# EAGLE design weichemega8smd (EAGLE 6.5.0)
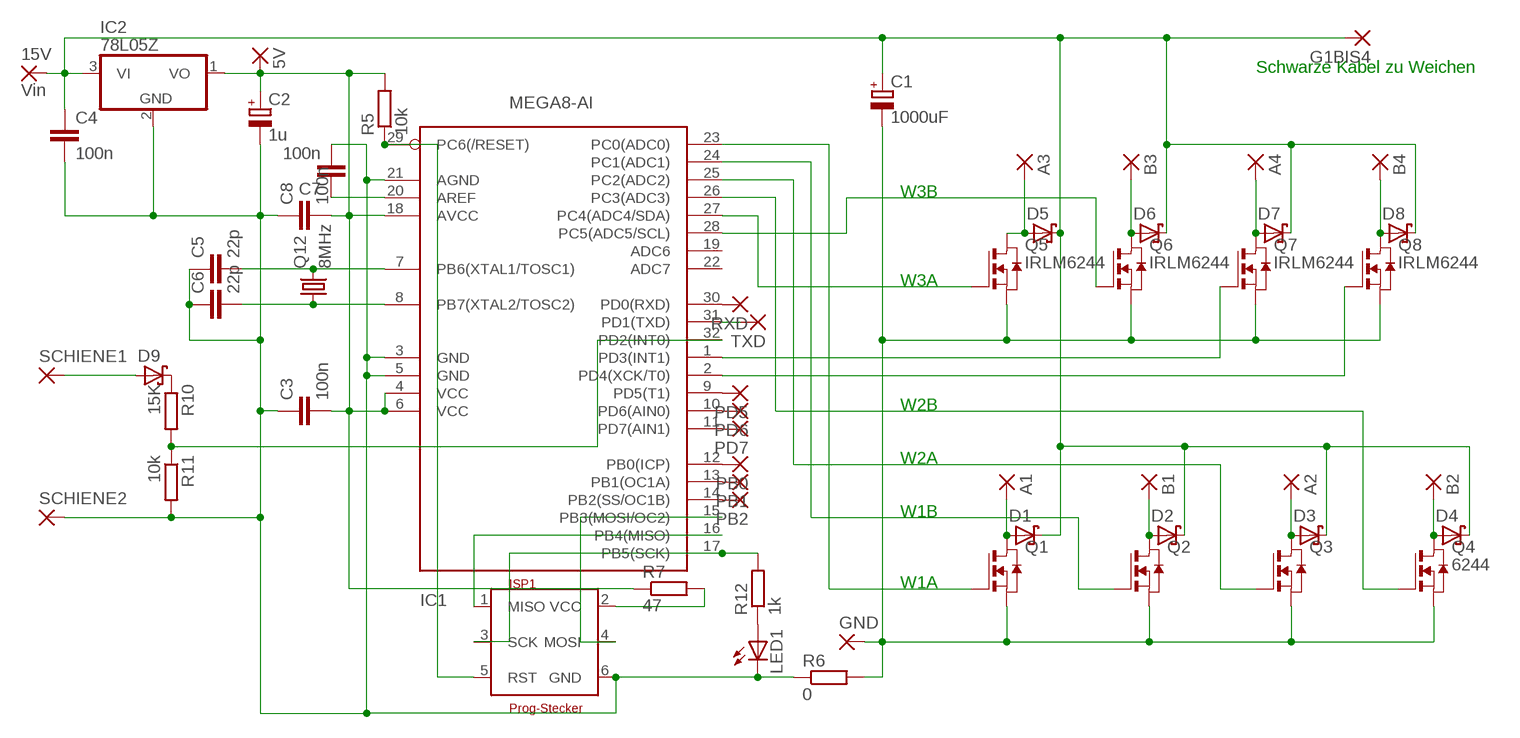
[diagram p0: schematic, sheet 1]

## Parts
5V  2,15/1,0  [2,15/1,0]
15V  Vin  2,15/1,0  [2,15/1,0]
A1  2,15/1,0  [2,15/1,0]
A2  2,15/1,0  [2,15/1,0]
A3  2,15/1,0  [2,15/1,0]
A4  2,15/1,0  [2,15/1,0]
B1  2,15/1,0  [2,15/1,0]
B2  2,15/1,0  [2,15/1,0]
B3  2,15/1,0  [2,15/1,0]
B4  2,15/1,0  [2,15/1,0]
C1  1000uF  CPOL-EUE2.5-7  [E2,5-7]
C2  1u  CPOL-EUE2.5-5  [E2,5-5]
C3  100n  C-EU025-024X044  [C025-024X044]
C4  100n  C-EU025-024X044  [C025-024X044]
C5  22p  C-EU025-024X044  [C025-024X044]
C6  22p  C-EU025-024X044  [C025-024X044]
C7  100n  C-EU025-024X044  [C025-024X044]
C8  100n  C-EU025-024X044  [C025-024X044]
D1  SCHOTTKY-DIODESMD  [SMB]
D2  SCHOTTKY-DIODESMD  [SMB]
D3  SCHOTTKY-DIODESMD  [SMB]
D4  SCHOTTKY-DIODESMD  [SMB]
D5  SCHOTTKY-DIODESMD  [SMB]
D6  SCHOTTKY-DIODESMD  [SMB]
D7  SCHOTTKY-DIODESMD  [SMB]
D8  SCHOTTKY-DIODESMD  [SMB]
D9  SCHOTTKY-DIODESMD  [SMB]
G1BIS4  2,15/1,0  [2,15/1,0]
GND  2,15/1,0  [2,15/1,0]
IC1  MEGA8-AI  [TQFP32-08]
IC2  78L05Z  [TO92]
ISP1  Prog-Stecker  ISP6N  [ISP6]
LED1  TLLG4400  [LED3MM]
PB0  1,6/0,8  [1,6/0,8]
PB1  1,6/0,8  [1,6/0,8]
PB2  1,6/0,8  [1,6/0,8]
PD5  1,6/0,8  [1,6/0,8]
PD6  1,6/0,8  [1,6/0,8]
PD7  1,6/0,8  [1,6/0,8]
Q1  NMOSSOT23  [SOT-23]
Q2  NMOSSOT23  [SOT-23]
Q3  NMOSSOT23  [SOT-23]
Q4  6244  NMOSSOT23  [SOT-23]
Q5  IRLM6244  NMOSSOT23  [SOT-23]
Q6  IRLM6244  NMOSSOT23  [SOT-23]
Q7  IRLM6244  NMOSSOT23  [SOT-23]
Q8  IRLM6244  NMOSSOT23  [SOT-23]
Q12  8MHz  CRYSTALTC26V  [TC26V]
R5  10k  R-EU_M1406  [M1406]
R6  0  R-EU_0204/5  [0204/5]
R7  47  R-EU_0204/5  [0204/5]
R10  15K  R-EU_M1406  [M1406]
R11  10k  R-EU_M1406  [M1406]
R12  1k  R-EU_0204/2V  [0204V]
RXD  1,6/0,8  [1,6/0,8]
SCHIENE1  2,15/1,0  [2,15/1,0]
SCHIENE2  2,15/1,0  [2,15/1,0]
TXD  1,6/0,8  [1,6/0,8]

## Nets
GND [dick]: C2.- C3.1 C4.2 C5.1 C6.1 C7.2 C8.1 IC1.3(GND) IC1.5(GND) IC1.21(AGND) IC2.2(GND) ISP1.6(GND) LED1.K(C) R6.1 R11.2 SCHIENE2.1(P)
GND1 [dick3]: C1.- GND.1(P) Q1.2(S) Q2.2(S) Q3.2(S) Q4.2(S) Q5.2(S) Q6.2(S) Q7.2(S) Q8.2(S) R6.2
N$1: IC1.23(PC0(ADC0)) Q1.3(G)
N$2: IC1.26(PC3(ADC3)) Q4.3(G)
N$3: IC1.24(PC1(ADC1)) Q2.3(G)
N$4: IC1.25(PC2(ADC2)) Q3.3(G)
N$5: IC1.28(PC5(ADC5/SCL)) Q6.3(G)
N$6: IC1.16(PB4(MISO)) ISP1.1(MISO)
N$7 [dick2]: B2.1(P) D4.A Q4.1(D)
N$8: IC1.10(PD6(AIN0)) PD6.1(P)
N$9: IC1.29(PC6(/RESET)) ISP1.5(RST) R5.1
N$10 [dick2]: A1.1(P) D1.A Q1.1(D)
N$11 [dick2]: B1.1(P) D2.A Q2.1(D)
N$12 [dick2]: A2.1(P) D3.A Q3.1(D)
N$13 [dick2]: A4.1(P) D7.A Q7.1(D)
N$14: IC1.15(PB3(MOSI/OC2)) ISP1.4(MOSI)
N$15 [dick2]: A3.1(P) D5.A Q5.1(D)
N$16 [dick2]: B3.1(P) D6.A Q6.1(D)
N$17: LED1.A R12.1
N$18: IC1.17(PB5(SCK)) ISP1.3(SCK) R12.2
N$19: IC1.11(PD7(AIN1)) PD7.1(P)
N$20 [dick2]: D9.C R10.1
N$21: C5.2 IC1.7(PB6(XTAL1/TOSC1)) Q12.2
N$22: C6.2 IC1.8(PB7(XTAL2/TOSC2)) Q12.1
N$23 [dick]: ISP1.2(VCC) R7.2
N$24 [dick2]: D9.A SCHIENE1.1(P)
N$25: IC1.32(PD2(INT0)) R10.2 R11.1
N$26 [dick2]: B4.1(P) D8.A Q8.1(D)
N$27: C7.1 IC1.20(AREF)
N$28: IC1.30(PD0(RXD)) RXD.1(P)
N$29: IC1.31(PD1(TXD)) TXD.1(P)
N$30: IC1.12(PB0(ICP)) PB0.1(P)
N$31: IC1.13(PB1(OC1A)) PB1.1(P)
N$32: IC1.14(PB2(SS/OC1B)) PB2.1(P)
N$33: IC1.27(PC4(ADC4/SDA)) Q5.3(G)
N$34: IC1.1(PD3(INT1)) Q7.3(G)
N$35: IC1.2(PD4(XCK/T0)) Q8.3(G)
N$36: IC1.9(PD5(T1)) PD5.1(P)
VCC [dick]: 5V.1(P) C2.+ C3.2 C8.2 IC1.4(VCC) IC1.6(VCC) IC1.18(AVCC) IC2.1(VO) R5.2 R7.1
VIN [dick3]: 15V.1(P) C1.+ C4.1 D1.C D2.C D3.C D4.C D5.C D6.C D7.C D8.C G1BIS4.1(P) IC2.3(VI)
Unconnected: IC1.19(ADC6) IC1.22(ADC7)

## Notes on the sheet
- Schwarze Kabel zu Weichen
- W3B
- W3A
- W2B
- W2A
- W1B
- W1A

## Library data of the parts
5V 15V A1-A4 B1-B4 G1BIS4 GND SCHIENE1 SCHIENE2 = wirepad:2,15/1,0: THROUGH-HOLE PAD
C1 C2 = rcl:CPOL-EU: POLARIZED CAPACITOR, European symbol
C3-C8 = rcl:C-EU: CAPACITOR, European symbol
D1-D9 = diode:SCHOTTKY-DIODE: Schottky Diode
IC1 = avr-7:MEGA8: MICROCONTROLLER 8 Kbytes FLASH 1 kbytes SRAM 512 bytes EEPROM USART 6-channel 10 bit ADC 2-channel 8 bit ADC
IC2 = linear:78*: Positive VOLTAGE REGULATOR Source: http://cache.national.com/ds/LM/LM78L05.pdf http://www.fairchildsemi.com/ds/LM/LM7805.pdf
ISP1 = 6_stecker:ISP6: ISP-Stecker 6polig
LED1 = led:TLLG4400: Low Current (2mA) LED 3 mm Tinted Diffused Package color GREEN; MF: VISHAY SEMICONDUCTOR; OC_FARNELL: 1612435
PB0 PB1 PB2 PD5-PD7 RXD TXD = wirepad:1,6/0,8: THROUGH-HOLE PAD
Q1-Q8 = zetex:NMOSSOT23: MOS FET; OC_FARNELL: unknown; OC_NEWARK: unknown
Q12 = crystal:CRYSTAL: CRYSTAL; OC_FARNELL: unknown; OC_NEWARK: unknown
R5-R7 R10-R12 = rcl:R-EU_: RESISTOR, European symbol

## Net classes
0 default: width 0.254 mm
1 dick: width 0.406 mm
2 dick2: width 0.813 mm
3 dick3: width 1.016 mm

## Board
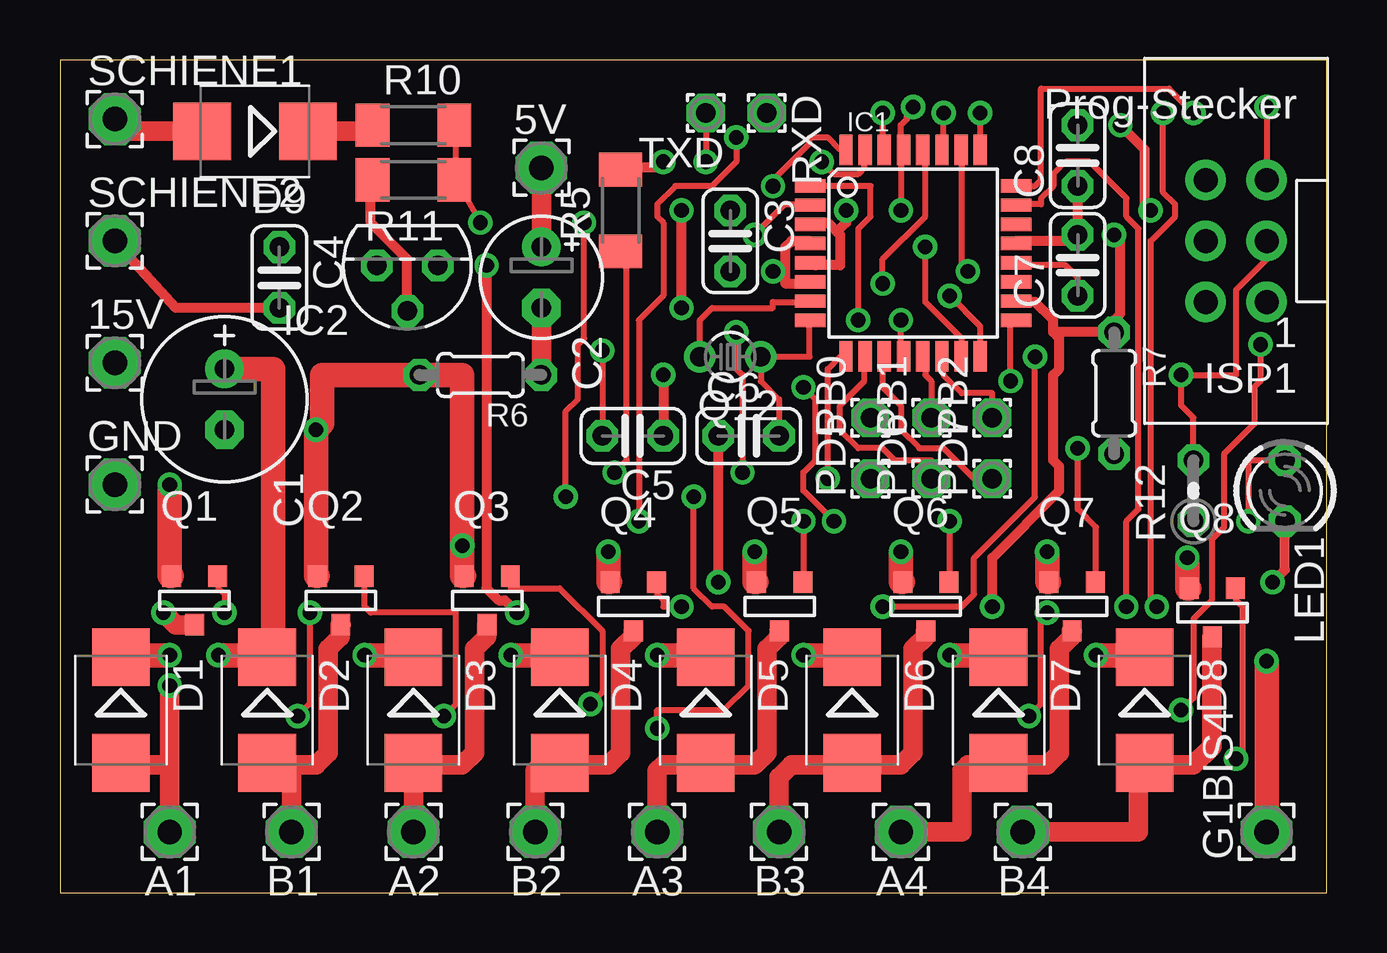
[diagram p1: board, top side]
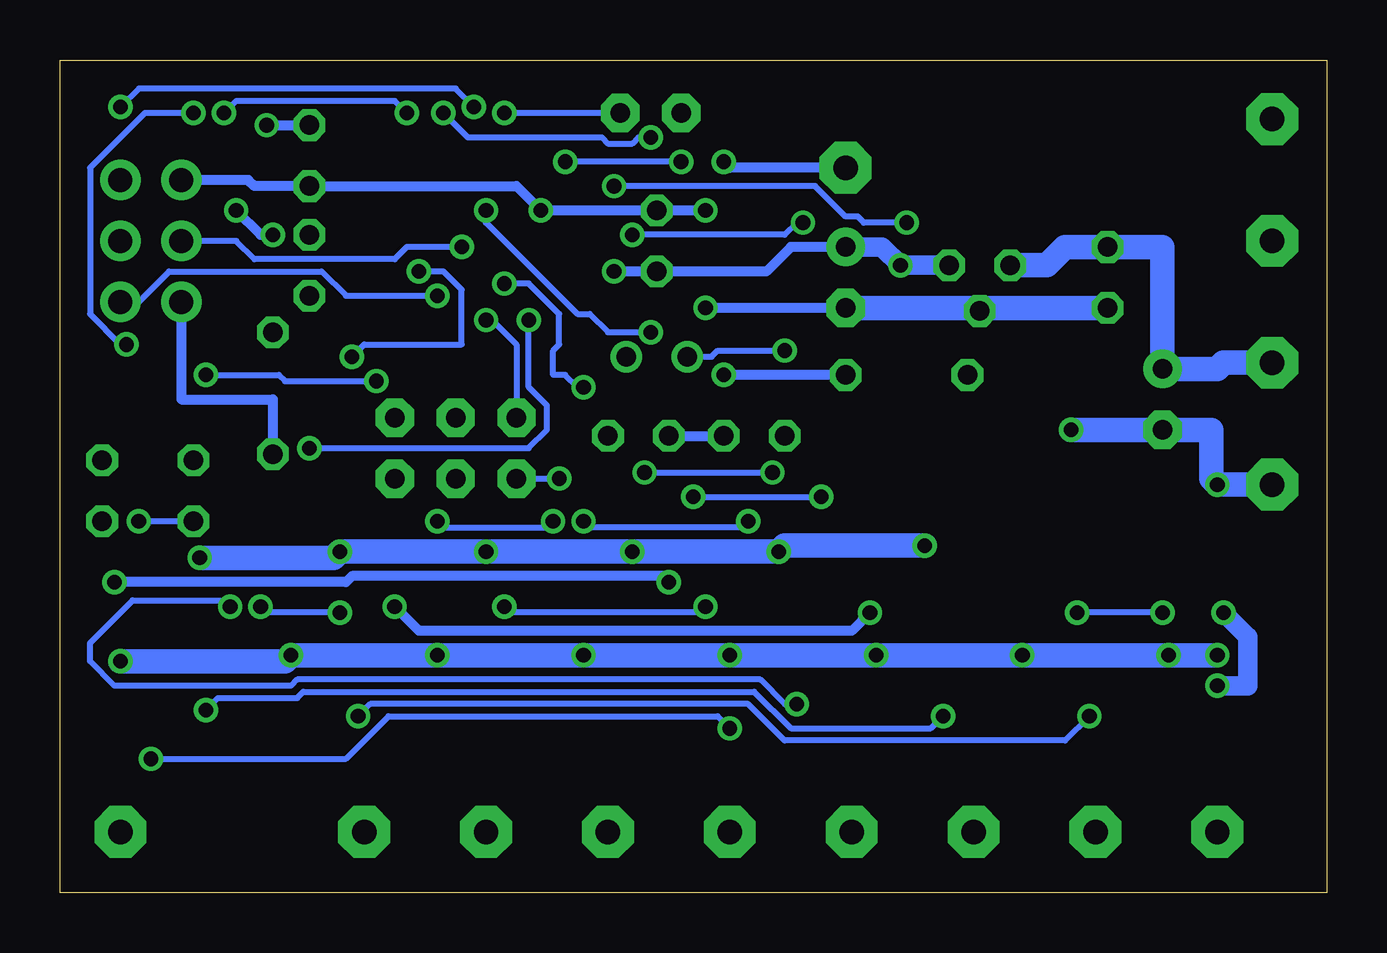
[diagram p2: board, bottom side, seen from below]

Size 52.81 x 34.72 mm. Coordinates in mm from the lower left corner, seen from the top.
Outline: 0,0 52.81,0 52.81,34.72 0,34.72 0,0
Copper layers (1*16): Top 0.035mm / dielectric 1.5mm / Bottom 0.035mm
Design rules "default": minimum track width 10mil, minimum drill 24mil, track to track 8mil, track to pad 8mil, pad to pad 8mil, via to via 8mil, smd to smd 8mil, copper to edge 40mil, drill to drill 8mil, minimum pad ring 10mil, minimum via ring 8mil, stop-mask expansion 4mil, vias tented up to drill 0mil, thermal gap 10mil

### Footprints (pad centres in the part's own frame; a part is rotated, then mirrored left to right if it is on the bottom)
2,15/1,0 = drill 1.016 pad 2.159 octagon: 1 0,0
E2,5-7 = drill 0.813 pad 1.6: + -1.27,0 | drill 0.813 pad 1.6 octagon: - 1.27,0
E2,5-5 = drill 0.813 pad 1.6: + -1.27,0 | drill 0.813 pad 1.6 octagon: - 1.27,0
C025-024X044 = drill 0.813 octagon: 1 -1.27,0; 2 1.27,0
SMB = smd 2.4 x 2.4: A 2.2,0; C -2.2,0
TQFP32-08 = smd 1.27 x 0.559: 1 -4.293,2.8; 2 -4.293,2; 3 -4.293,1.2; 4 -4.293,0.4; 5 -4.293,-0.4; 6 -4.293,-1.2; 7 -4.293,-2; 8 -4.293,-2.8; 17 4.293,-2.8; 18 4.293,-2; 19 4.293,-1.2; 20 4.293,-0.4; 21 4.293,0.4; 22 4.293,1.2; 23 4.293,2; 24 4.293,2.8 | smd 0.559 x 1.27: 9 -2.8,-4.293; 10 -2,-4.293; 11 -1.2,-4.293; 12 -0.4,-4.293; 13 0.4,-4.293; 14 1.2,-4.293; 15 2,-4.293; 16 2.8,-4.293; 25 2.8,4.293; 26 2,4.293; 27 1.2,4.293; 28 0.4,4.293; 29 -0.4,4.293; 30 -1.2,4.293; 31 -2,4.293; 32 -2.8,4.293
TO92 = drill 0.813 octagon: 1 -1.27,0; 2 0,1.905; 3 1.27,0
ISP6 = drill 1 pad 1.676: 1 -1.27,2.54; 2 1.27,2.54; 3 -1.27,0; 4 1.27,0; 5 -1.27,-2.54; 6 1.27,-2.54
LED3MM = drill 0.813 octagon: A -1.27,0; K 1.27,0
1,6/0,8 = drill 0.813 pad 1.6 octagon: 1 0,0
SOT-23 = smd 0.787 x 0.889: 1 0.025,-1.016; 2 -0.94,1.016; 3 0.991,1.016
TC26V = drill 0.813: 1 -1.27,0; 2 1.27,0
M1406 = smd 1.4 x 1.8: 1 -1.7,0; 2 1.7,0
0204/5 = drill 0.813 octagon: 1 -2.54,0; 2 2.54,0
0204V = drill 0.813 octagon: 1 -1.27,0; 2 1.27,0

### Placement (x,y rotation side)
5V  20.07,30.23 0 top
15V  2.29,22.1 0 top
A1  4.57,2.54 180 top
A2  14.73,2.54 180 top
A3  24.89,2.54 180 top
A4  35.05,2.54 180 top
B1  9.65,2.54 180 top
B2  19.81,2.54 180 top
B3  29.97,2.54 180 top
B4  40.13,2.54 180 top
C1  6.86,20.57 270 top
C2  20.07,25.65 270 top
C3  27.94,27.18 270 top
C4  9.14,25.65 270 top
C5  23.88,19.05 180 top
C6  28.7,19.05 0 top
C7  42.42,26.16 90 top
C8  42.42,30.73 90 top
D1  2.54,7.62 270 top
D2  8.64,7.62 270 top
D3  14.73,7.62 270 top
D4  20.83,7.62 270 top
D5  26.92,7.62 270 top
D6  33.02,7.62 270 top
D7  39.12,7.62 270 top
D8  45.21,7.62 270 top
D9  8.13,31.75 180 top
G1BIS4  50.29,2.54 90 top
GND  2.29,17.02 0 top
IC1  35.56,26.67 0 top
IC2  14.48,26.16 180 top
ISP1  49.02,27.18 180 top
LED1  51.05,16.76 270 top
PB0  33.78,19.81 90 top
PB1  36.32,19.81 90 top
PB2  38.86,19.81 90 top
PD5  33.78,17.27 90 top
PD6  36.32,17.27 90 top
PD7  38.86,17.27 90 top
Q1  5.59,12.19 0 top
Q2  11.68,12.19 0 top
Q3  17.78,12.19 0 top
Q4  23.88,11.94 0 top
Q5  29.97,11.94 0 top
Q6  36.07,11.94 0 top
Q7  42.16,11.94 0 top
Q8  48.01,11.68 0 top
Q12  27.94,22.35 180 top
R5  23.37,28.45 90 top
R6  17.53,21.59 180 top
R7  43.94,20.83 270 top
R10  14.73,32 0 top
R11  14.73,29.72 180 top
R12  47.24,16.76 90 top
RXD  29.46,32.51 270 top
SCHIENE1  2.29,32.26 0 top
SCHIENE2  2.29,27.18 0 top
TXD  26.92,32.51 180 top

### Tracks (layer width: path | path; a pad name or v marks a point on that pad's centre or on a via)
GND  (via drill 0.61)
  Top 0.406: LED1.K 51.05,13.46 v50.55,12.95 | C6.1 v27.43,12.95 | 32.38,27.56 32,27.94 31.5,27.94 IC1.3 | 32.38,27.56 32.51,27.43 32.51,26.16 31.5,26.16 IC1.5 | 32.38,27.56 32.77,27.94 v32.77,28.45 | IC1.21 39.88,27.18 42.42,27.18 C7.2 C8.1 | IC2.2 14.48,26.42 12.95,27.94 12.95,29.72 R11.2 | SCHIENE2.1 4.83,24.38 C4.2 | v25.91,24.38 v25.91,28.45 | v25.15,21.59 C5.1
  Top 0.813: C2.- R6.1
  Bottom 0.406: C6.1 C5.1 | v50.55,12.95 40.89,12.95 40.64,13.21 27.69,13.21 v27.43,12.95 | ISP1.6 44.96,29.72 44.7,29.46 C8.1 33.78,29.46 v32.77,28.45 C3.1 v25.91,28.45 | 14.48,24.38 IC2.2 | C2.- v25.91,24.38 | R6.1 v25.15,21.59
  Bottom 1.016: C4.2 14.48,24.38 C2.-
GND1  (via drill 0.61)
  Top 1.016: v22.86,14.22 22.86,12.95 Q4.2 | v28.96,14.22 28.96,12.95 Q5.2 | v35.05,14.22 35.05,12.95 Q6.2 | v41.15,14.22 41.15,12.95 Q7.2 | v46.99,13.97 46.99,12.7 Q8.2 | Q3.2 16.76,13.21 v16.76,14.48 16.76,21.59 R6.2 10.92,21.59 10.92,19.56 v10.67,19.3 10.67,13.21 Q2.2 | v4.57,17.02 4.57,13.21 Q1.2
  Bottom 1.016: v46.99,13.97 41.4,13.97 v41.15,14.22 v35.05,14.22 v28.96,14.22 v22.86,14.22 22.61,14.48 v16.76,14.48 | GND.1 v4.57,17.02 4.83,17.27 4.83,19.3 C1.- v10.67,19.3
N$1  (via drill 0.61)
  Top 0.254: v44.45,11.94 44.45,15.49 44.96,16 44.96,27.69 44.45,28.19 44.45,28.96 42.93,30.48 41.91,30.48 41.4,29.97 41.4,29.46 40.89,28.96 40.89,28.7 39.88,28.7 IC1.23 | v41.15,11.68 40.89,11.43 40.89,7.87 v40.39,7.37 | v9.91,7.37 10.41,7.87 v10.41,11.68 | v6.86,11.68 6.86,12.45 6.6,12.7 6.6,13.21 Q1.3
  Bottom 0.254: v44.45,11.94 44.2,11.68 v41.15,11.68 | v40.39,7.37 39.88,7.87 24.13,7.87 22.61,6.35 10.92,6.35 v9.91,7.37 | v6.86,11.68 v10.41,11.68
N$2  (via drill 0.61)
  Top 0.254: v37.85,25.91 37.59,26.16 37.59,30.73 IC1.26 | v40.64,22.35 40.64,16.51 38.1,13.97 38.1,12.45 37.59,11.94 v34.29,11.94 | v25.91,11.94 25.15,11.94 25.15,12.19 24.89,12.45 24.89,12.95 Q4.3
  Bottom 0.254: v37.85,25.91 36.83,25.91 36.07,25.15 36.07,22.86 40.13,22.86 v40.64,22.35 | v34.29,11.94 34.04,11.68 26.16,11.68 v25.91,11.94
N$3  (via drill 0.61)
  Top 0.254: v16,7.37 16.51,7.87 16.51,11.68 12.95,11.68 12.7,11.94 12.7,13.21 Q2.3 | v46.74,7.62 47.24,8.13 47.24,11.43 48.01,12.19 48.01,14.73 48.51,15.24 48.51,18.29 49.78,19.56 49.78,21.08 50.04,21.34 v50.04,22.86 | v47.24,32.51 46.23,33.53 40.89,33.53 40.89,29.72 40.64,29.46 39.88,29.46 IC1.24
  Bottom 0.254: v16,7.37 16.51,6.86 22.35,6.86 23.88,8.38 42.67,8.38 42.93,8.13 46.23,8.13 v46.74,7.62 | v50.04,22.86 50.29,22.86 51.56,24.13 51.56,30.23 49.28,32.51 v47.24,32.51
N$4  (via drill 0.61)
  Top 0.254: v38.35,32.51 38.35,30.99 IC1.25 | v45.97,32.51 45.97,29.21 46.48,28.7 46.48,28.19 45.47,27.18 45.47,12.19 v45.72,11.94 | v22.1,7.87 22.61,8.38 22.61,10.92 20.83,12.7 18.8,12.7 18.8,13.21 Q3.3
  Bottom 0.254: v38.35,32.51 38.86,33.02 45.47,33.02 v45.97,32.51 | v45.72,11.94 45.97,12.19 49.78,12.19 51.56,10.41 51.56,9.65 50.55,8.64 43.18,8.64 42.93,8.89 23.62,8.89 22.61,7.87 v22.1,7.87
N$5  (via drill 0.61)
  Top 0.254: v34.29,25.4 34.29,26.42 36.07,28.19 36.07,30.73 IC1.28 | v30.99,21.08 31.5,20.57 31.5,18.03 30.99,17.53 30.99,16.76 v32.26,15.49 | v37.08,15.49 37.08,12.95 Q6.3
  Bottom 0.254: v34.29,25.4 33.27,25.4 32,24.13 32,22.86 32.26,22.61 32.26,21.59 31.75,21.59 31.24,21.08 v30.99,21.08 | v32.26,15.49 32.51,15.24 36.83,15.24 v37.08,15.49
N$6  (via drill 0.61)
  Top 0.254: v37.08,24.89 38.35,23.62 38.35,22.61 IC1.16
  Bottom 0.254: v37.08,24.89 40.89,24.89 41.91,25.91 48.26,25.91 49.53,24.64 ISP1.1
N$7
  Top 0.813: Q4.1 23.88,10.92 23.88,10.67 23.37,10.16 23.37,5.84 22.86,5.33 20.83,5.33 D4.A 20.57,5.33 20.07,5.33 19.81,5.08 B2.1
N$8
  Top 0.254: PD6.1 36.32,18.03 34.8,18.03 34.29,18.54 33.27,18.54 32.51,19.3 32.51,20.32 33.53,21.34 33.53,22.35 IC1.10
N$9  (via drill 0.61)
  Top 0.254: v50.29,32.77 ISP1.5 | v35.56,32.77 35.31,32.51 35.31,32.26 35.05,32 35.05,30.99 IC1.29 35.05,30.73 v35.05,28.45 | v23.11,17.53 23.62,18.03 23.62,26.67 23.37,26.67 R5.1 | v28.45,17.53 28.45,21.59 28.19,21.84 v28.19,23.37
  Bottom 0.254: v50.29,32.77 49.53,33.53 36.32,33.53 v35.56,32.77 | v28.45,17.53 v23.11,17.53 | v28.19,23.37 29.97,23.37 30.73,24.13 31.24,24.13 35.05,27.94 v35.05,28.45
N$10  (via drill 0.61)
  Top 0.813: Q1.1 4.83,11.18 v4.32,11.68 | A1.1 4.57,5.33 | 4.57,5.33 v4.57,8.64 | 4.57,5.33 2.54,5.33 D1.A
  Bottom 0.813: v4.32,11.68 3.3,10.67 3.3,8.64 v4.57,8.64
N$11
  Top 0.813: Q2.1 11.68,11.18 11.68,10.67 11.18,10.16 11.18,5.84 10.67,5.33 8.64,5.33 D2.A 9.65,5.08 B1.1
N$12
  Top 0.813: Q3.1 17.78,11.18 17.78,10.67 17.27,10.16 17.27,5.84 16.76,5.33 14.73,5.33 D3.A A2.1
N$13
  Top 0.813: Q7.1 42.16,10.92 42.16,10.67 41.66,10.16 41.66,5.84 41.15,5.33 39.12,5.33 D7.A 38.86,5.33 37.85,5.33 37.59,5.08 37.59,2.54 A4.1
N$14  (via drill 0.61)
  Top 0.254: v36.07,26.92 36.07,24.64 37.59,23.11 37.59,22.61 IC1.15
  Bottom 0.254: ISP1.4 45.47,27.18 44.7,26.42 38.86,26.42 38.35,26.92 v36.07,26.92
N$15
  Top 0.813: Q5.1 29.97,10.92 29.97,10.67 29.46,10.16 29.46,5.84 28.96,5.33 26.92,5.33 D5.A 26.67,5.33 25.15,5.33 24.89,5.08 A3.1
N$16
  Top 0.813: Q6.1 36.07,10.92 36.07,10.67 35.56,10.16 35.56,5.84 35.05,5.33 33.02,5.33 D6.A 32.77,5.33 30.48,5.33 29.97,4.83 B3.1
N$17  (via drill 0.61)
  Top 0.254: v49.53,15.49 49.53,18.03 LED1.A
  Bottom 0.254: v49.53,15.49 R12.1
N$18  (via drill 0.61)
  Top 0.254: v39.62,21.34 39.62,23.62 IC1.17 | R12.2 47.24,19.81 46.74,20.32 v46.74,21.59 49.02,21.59 49.02,25.15 50.29,26.42 ISP1.3
  Bottom 0.254: v39.62,21.34 43.43,21.34 43.69,21.59 v46.74,21.59
N$19
  Top 0.254: PD7.1 38.1,17.27 36.83,18.54 35.81,18.54 35.05,19.3 35.05,20.32 34.29,21.08 34.29,22.35 IC1.11
N$20
  Top 0.813: R10.1 12.7,32 12.45,31.75 D9.C
N$21  (via drill 0.61)
  Top 0.254: Q12.2 26.67,23.88 27.18,24.38 29.72,24.38 29.72,24.64 31.24,24.64 IC1.7 | v22.61,22.61 C5.2
  Bottom 0.254: v22.61,22.61 25.4,22.61 25.65,22.35 Q12.2
N$22
  Top 0.254: IC1.8 31.24,23.62 31.24,22.35 Q12.1 29.21,21.34 29.97,20.57 C6.2
N$23
  Bottom 0.406: R7.2 43.94,20.57 47.75,20.57 ISP1.2
N$24
  Top 0.813: D9.A 2.29,31.75 SCHIENE1.1
N$25  (via drill 0.61)
  Top 0.254: 16.51,29.72 16.51,32 R10.2 | v29.72,29.46 29.72,29.72 31.24,31.24 31.24,31.5 32,31.5 32.51,30.99 IC1.32 | 16.51,29.72 v17.53,27.94 | 16.51,29.72 R11.1
  Bottom 0.254: v29.72,29.46 21.34,29.46 20.07,28.19 19.56,28.19 19.3,27.94 v17.53,27.94
N$26
  Top 0.813: Q8.1 48.01,10.67 48.01,6.1 47.24,5.33 45.21,5.33 D8.A 44.96,5.08 44.96,2.54 B4.1
N$27
  Top 0.254: C7.1 42.42,25.65 41.91,26.16 39.88,26.16 IC1.20
N$28  (via drill 0.61)
  Top 0.254: v34.29,32.51 34.29,30.99 IC1.30
  Bottom 0.254: RXD.1 v34.29,32.51
N$29  (via drill 0.61)
  Top 0.254: v31.75,30.48 32.26,29.97 33.27,29.97 33.53,30.23 33.53,30.73 IC1.31 | TXD.1 v26.92,30.48
  Bottom 0.254: v26.92,30.48 v31.75,30.48
N$30  (via drill 0.61)
  Top 0.254: v35.05,23.88 35.05,22.61 IC1.12
  Bottom 0.254: PB0.1 33.78,22.86 34.8,23.88 v35.05,23.88
N$31
  Top 0.254: PB1.1 36.32,21.34 36.07,21.59 36.07,22.35 IC1.13
N$32
  Top 0.254: PB2.1 38.86,20.83 37.59,20.83 36.83,21.59 36.83,22.35 IC1.14
N$33  (via drill 0.61)
  Top 0.254: v30.99,15.49 30.99,12.95 Q5.3 | v24.13,15.49 24.13,23.88 25.15,24.89 25.15,27.94 24.89,28.19 24.89,28.7 25.65,29.46 27.18,29.46 28.19,30.48 v28.19,31.5 | v36.83,32.51 36.83,30.99 IC1.27
  Bottom 0.254: v30.99,15.49 30.73,15.24 24.38,15.24 v24.13,15.49 | v28.19,31.5 28.7,31.5 28.96,31.24 29.97,31.24 30.23,31.5 35.81,31.5 v36.83,32.51
N$34  (via drill 0.61)
  Top 0.254: v33.27,23.88 33.27,27.69 33.78,28.19 33.78,29.46 31.5,29.46 IC1.1 | v42.42,18.54 42.42,16 43.18,15.24 43.18,12.95 Q7.3
  Bottom 0.254: v33.27,23.88 33.27,21.08 32.51,20.32 32.51,19.3 33.27,18.54 v42.42,18.54
N$35  (via drill 0.61)
  Top 0.254: v28.96,27.43 30.23,28.7 31.24,28.7 IC1.2 | v21.84,27.94 21.84,23.11 21.59,22.86 21.59,20.57 21.08,20.07 v21.08,16.51 | v26.42,16.51 26.42,12.7 27.18,11.94 27.69,11.94 28.7,10.92 28.7,8.64 27.69,7.62 24.89,7.62 v24.89,6.86 | v49.02,5.59 49.28,5.84 49.28,11.94 49.02,12.19 49.02,12.7 Q8.3
  Bottom 0.254: v28.96,27.43 22.61,27.43 22.1,27.94 v21.84,27.94 | v26.42,16.51 v21.08,16.51 | v24.89,6.86 25.4,7.37 39.12,7.37 40.89,5.59 v49.02,5.59
N$36  (via drill 0.61)
  Top 0.254: v32,17.27 32,21.84 32.51,22.35 IC1.9
  Bottom 0.254: PD5.1 v32,17.27
VCC  (via drill 0.61)
  Top 0.406: 41.4,23.37 41.4,23.88 40.64,24.64 39.88,24.64 IC1.18 | 41.4,23.37 R7.1 43.94,23.88 44.2,24.13 44.2,27.18 v43.94,27.43 | v44.2,32 45.21,30.99 45.21,28.7 v45.47,28.45 | 30.23,25.91 30.23,26.92 30.48,27.18 31.24,27.18 IC1.4 | 30.23,25.91 30.23,25.4 31.24,25.4 IC1.6 | v29.72,25.91 30.23,25.91 | v25.15,30.48 25.15,30.23 23.37,30.23 R5.2 | 41.4,23.37 41.66,23.11 41.66,21.84 41.4,21.59 41.4,18.03 41.66,17.78 41.66,16.76 38.86,13.97 v38.86,11.94 | v19.05,11.68 18.54,12.19 18.29,12.19 17.78,12.7 v17.78,26.16
  Top 0.813: 5V.1 C2.+
  Bottom 0.406: v44.2,32 C8.2 | v45.47,28.45 44.45,27.43 v43.94,27.43 | v29.72,25.91 C3.2 23.37,25.91 22.35,26.92 C2.+ | v25.15,30.48 24.89,30.23 5V.1 | v38.86,11.94 37.85,10.92 19.81,10.92 v19.05,11.68
  Bottom 0.813: IC2.1 v17.78,26.16 18.54,26.92 C2.+
VIN  (via drill 0.61)
  Top 1.016: v4.57,9.91 2.54,9.91 D1.C | v6.6,9.91 8.64,9.91 D2.C 8.89,10.16 8.89,21.84 C1.+ | v12.7,9.91 14.73,9.91 D3.C | v18.8,9.91 20.83,9.91 D4.C | v24.89,9.91 26.92,9.91 D5.C | v30.99,9.91 33.02,9.91 D6.C | v37.08,9.91 39.12,9.91 D7.C | v43.18,9.91 45.21,9.91 D8.C | v50.29,9.65 G1BIS4.1
  Bottom 1.016: IC2.3 11.68,26.16 10.92,26.92 C4.1 6.86,26.92 C1.+ 4.57,21.84 4.32,22.1 15V.1 | v4.57,9.91 v6.6,9.91 v12.7,9.91 v18.8,9.91 v24.89,9.91 v30.99,9.91 v37.08,9.91 v43.18,9.91 43.43,9.65 v50.29,9.65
